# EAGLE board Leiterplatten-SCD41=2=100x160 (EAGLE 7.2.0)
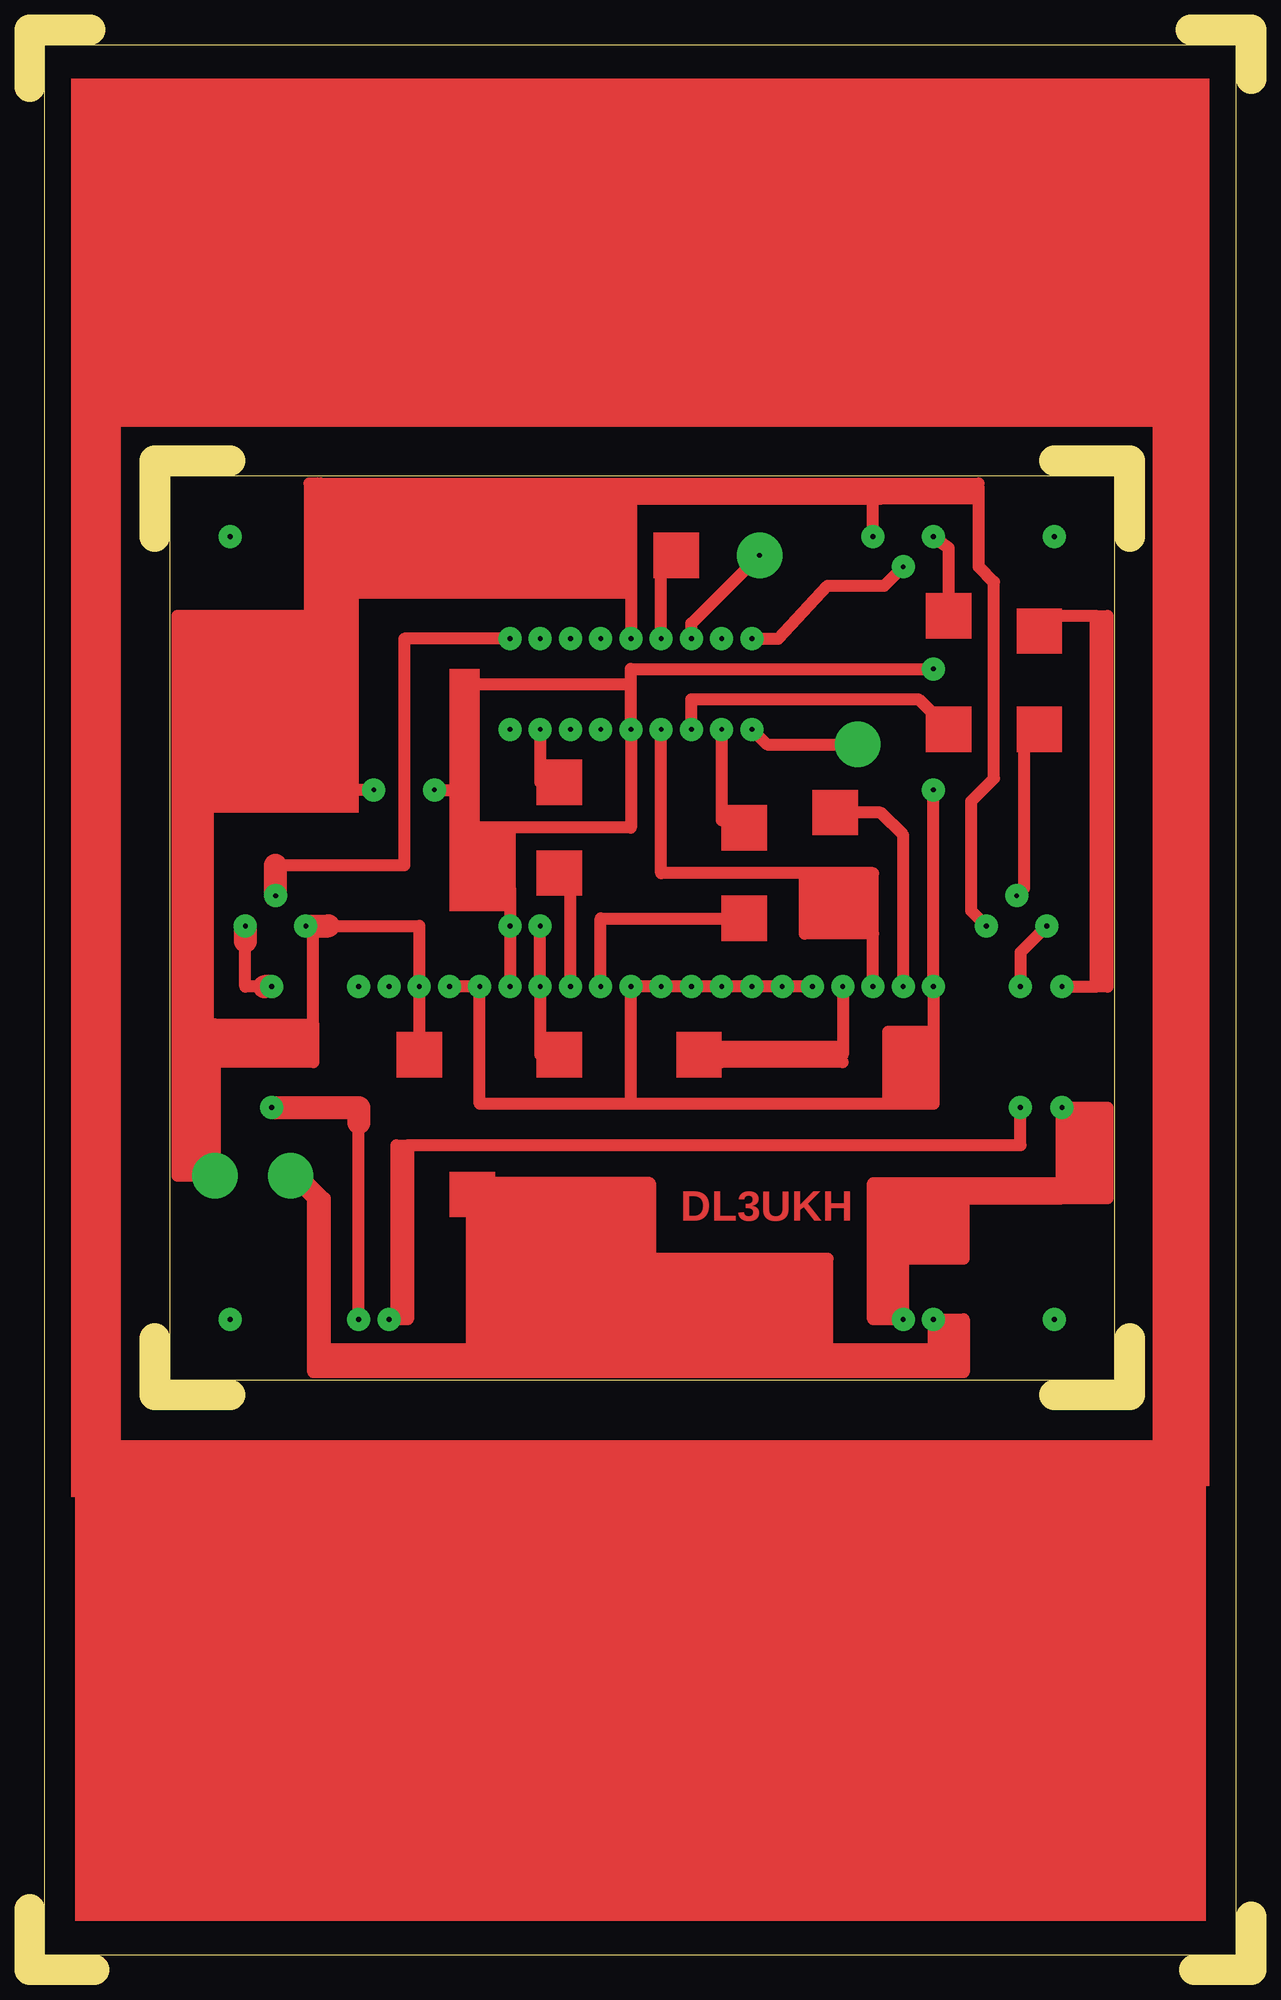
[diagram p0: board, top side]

Size 102.55 x 162.88 mm. Coordinates in mm from the lower left corner, seen from the top.
Outline: 5.4,0 0.32,0
Outline: 0,0 0,5.08
Outline: 97.79,0 102.55,0 102.55,4.45
Outline: 5.08,162.88 0,162.88 0,158.12
Outline: 102.55,158.75 102.55,162.88
Outline: 97.47,162.88 102.23,162.88
Outline: 10.48,120.33 10.48,126.68 16.83,126.68
Outline: 10.48,53.02 10.48,48.26 16.83,48.26
Outline: 86.04,48.26 92.39,48.26 92.39,53.02
Outline: 92.39,120.33 92.39,126.68 86.04,126.68
Outline: 1.27,1.27 101.28,1.27 101.28,161.61 1.27,161.61 1.27,1.27
Outline: 11.75,125.41 11.75,49.53 91.12,49.53 91.12,125.41 11.75,125.41
Copper layers (1*16): Top 0.035mm / dielectric 1.5mm / Bottom 0.035mm
Design rules "default": minimum track width 10mil, minimum drill 24mil, track to track 8mil, track to pad 8mil, pad to pad 8mil, via to via 8mil, smd to smd 8mil, copper to edge 40mil, drill to drill 8mil, minimum pad ring 10mil, minimum via ring 8mil, stop-mask expansion 4mil, vias tented up to drill 0mil, thermal gap 10mil

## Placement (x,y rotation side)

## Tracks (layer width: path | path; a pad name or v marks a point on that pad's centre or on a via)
S$1  (via drill 0.4 pad 1.93)
  Top 1.016: v33.97,99.06 36.51,99.06
S$2  (via drill 0.4 pad 1.93)
  other vias: 60.64,82.55
S$3  (via drill 0.4 pad 1.93)
  Top 1.016: v55.56,104.14 55.56,106.68 74.61,106.68 77.15,104.14
S$4  (via drill 0.4 pad 1.93)
  Top 1.016: v58.1,104.14 58.1,96.52 60.01,96.52
S$5  (via drill 0.4 pad 1.93)
  Top 1.016: v42.86,104.14 42.86,99.69 44.45,99.69
S$6  (via drill 0.4 pad 1.93)
  Top 1.016: v80.33,87.63 79.06,88.9 79.06,98.11 80.96,100.01 80.96,116.52 79.69,117.79 79.69,123.51 | 79.69,123.51 79.69,124.46 70.8,124.46 | 24.13,120.33 24.13,123.51 | 24.13,123.51 24.13,124.46 | 24.13,124.46 24.45,124.46 | 24.45,124.46 50.48,124.46 | 50.48,124.46 50.48,123.51 | 50.48,123.51 50.48,115.57 | 50.48,115.57 v50.48,111.76 | 50.48,124.46 58.42,124.46 | 58.42,124.46 70.8,124.46 | v70.8,120.33 70.8,124.46 | 58.42,124.46 71.44,123.51 | 24.13,124.46 24.13,124.78 | 24.13,124.78 24.45,124.78 | 24.45,124.78 79.69,124.78 | 50.48,123.51 24.13,123.51 | 50.48,123.51 71.44,123.51 | 79.69,123.51 71.44,123.51 | 24.45,124.46 24.45,124.78 | 24.13,124.78 23.5,124.78 23.5,112.39 | 50.48,115.57 23.81,115.57
S$7  (via drill 0.4 pad 1.93)
  other vias: 42.86,111.76
S$8  (via drill 0.4 pad 1.93)
  other vias: 86.04,54.61
S$9  (via drill 0.4 pad 1.93)
  other vias: 86.04,120.33
S$10  (via drill 0.01 pad 3.81, 0.4 pad 1.93)
  Top 1.016: v55.56,111.76 55.56,113.03 v61.28,118.74 | v60.64,104.14 61.91,102.87 v69.53,102.87 | v73.34,82.55 73.34,95.25 71.44,97.16 67.63,97.16
S$11  (via drill 0.4 pad 1.93)
  other vias: 58.1,82.55
S$12  (via drill 0.4 pad 1.93)
  Top 1.016: 31.75,69.21 83.19,69.21 v83.19,72.39 | 31.75,69.21 31.75,54.61 30.8,54.61 | 30.8,54.61 v30.16,54.61 | 30.8,54.61 30.8,69.21 31.75,69.21
S$13  (via drill 0.4 pad 1.93)
  other vias: 75.88,109.22
S$14  (via drill 0.4 pad 1.93)
  Top 1.016: v47.94,82.55 47.94,88.27 60.01,88.27
S$15  (via drill 0.4 pad 1.93)
  Top 1.016: v68.26,82.55 68.26,77.47 | 68.26,77.47 68.26,76.83 57.15,76.83 | 68.26,77.47 57.47,77.47
S$16  (via drill 0.4 pad 1.93)
  Top 1.016: v75.88,120.33 77.15,119.38 77.15,113.66
S$17  (via drill 0.4 pad 1.93)
  Top 1.016: v82.87,90.17 83.5,90.8 83.5,103.5
S$18  (via drill 0.4 pad 1.93)
  Top 1.016: 78.74,64.77 86.68,64.77 | 73.34,66.04 70.8,66.04 70.8,54.61 v73.34,54.61 73.34,59.69 | 73.34,66.04 78.42,66.04 | 78.42,66.04 86.68,66.04 | 86.68,66.04 v86.68,72.39 90.49,72.39 90.49,64.77 86.68,64.77 | 73.34,59.69 73.34,66.04 | 78.42,65.41 78.42,59.69 73.34,59.69 | 78.42,65.41 78.42,66.04 | 86.68,64.77 86.68,65.41 | 86.68,66.04 86.68,65.41 | 86.68,65.41 78.42,65.41
S$19  (via drill 0.4 pad 1.93)
  Top 1.016: v27.62,54.61 27.62,71.12
  Top 1.93: v20.32,72.39 27.62,72.39 27.62,71.12
S$20  (via drill 0.4 pad 1.93)
  Top 1.016: v28.89,99.06 24.77,99.06
S$21  (via drill 0.4 pad 1.93)
  other vias: 58.1,111.76
S$22  (via drill 0.4 pad 1.93)
  other vias: 40.32,104.14
S$23  (via drill 0.4 pad 1.93)
  Top 1.016: v75.88,99.06 v75.88,82.55 75.88,78.74 | 75.88,78.74 75.88,72.71 72.07,72.71 | 72.07,72.71 50.48,72.71 | v65.72,82.55 v63.18,82.55 v55.56,82.55 v50.48,82.55 50.48,72.71 | v35.24,82.55 v37.78,82.55 37.78,72.71 50.48,72.71 | 75.88,78.74 72.07,78.74 72.07,72.71
S$24  (via drill 0.4 pad 1.93)
  Top 1.016: v45.4,82.55 45.4,91.12
S$25  (via drill 0.4 pad 1.93)
  other vias: 30.16,82.55
S$26  (via drill 0.4 pad 1.93)
  other vias: 27.62,82.55
S$27  (via drill 0.4 pad 1.93)
  Top 1.016: v86.68,82.55 89.53,82.55 | 89.53,82.55 89.53,113.66 | 89.53,113.66 83.5,113.66 | 89.53,113.66 90.49,113.66 90.49,82.55 89.53,82.55
S$28  (via drill 0.01 pad 3.81, 0.4 pad 1.93)
  Top 1.016: 37.47,66.04 52.07,66.04 52.07,59.69 | 75.88,52.07 v75.88,54.61 78.42,54.61 78.42,50.8 | 75.88,52.07 75.88,50.8 | 75.88,50.8 37.15,50.8 | 37.15,50.8 37.15,59.69 | 37.15,59.69 37.15,65.09 | 37.15,50.8 23.81,50.8 | 23.81,50.8 23.81,52.07 | 23.81,52.07 23.81,64.77 | 23.81,64.77 v21.91,66.67 | 78.42,50.8 75.88,50.8 | 75.88,52.07 23.81,52.07 | 78.42,50.8 78.42,50.17 23.81,50.17 23.81,50.8 | 66.99,51.44 66.99,59.69 52.07,59.69 | 52.07,59.69 37.15,59.69 | 23.81,64.77 24.77,64.77 | 24.77,64.77 24.77,51.44 | 24.77,64.77 22.22,67.31
S$29  (via drill 0.4 pad 1.93)
  other vias: 16.83,54.61
S$30  (via drill 0.4 pad 1.93)
  Top 1.016: v40.32,111.76 31.43,111.76 31.43,92.71 20.64,92.71
  Top 1.93: v20.64,90.17 20.64,92.71
S$31  (via drill 0.4 pad 1.93)
  Top 1.016: v60.64,111.76 62.87,111.76 66.99,116.2 71.75,116.2 v73.34,117.79
S$32  (via drill 0.01 pad 3.81, 0.4 pad 1.93)
  Top 1.016: 24.13,113.66 24.13,110.49 14.92,110.49 | 24.13,113.66 14.92,113.66 | 14.92,113.66 12.38,113.66 12.38,79.38 | 14.92,113.66 14.92,110.49 | 12.38,79.38 12.38,66.67 v15.56,66.67 15.56,79.38 | 14.92,110.49 14.92,79.38 | 14.92,79.38 12.38,79.38 | 15.24,76.2 23.81,76.2 23.81,79.38 | 14.92,79.38 15.56,79.38 | 15.56,79.38 23.81,79.38 | 23.81,79.38 23.81,86.99 v23.18,87.63 | 25.08,87.63 32.7,87.63 v32.7,82.55 32.7,77.15 | 24.13,113.66 24.13,115.89
  Top 1.93: v23.18,87.63 25.08,87.63
S$33  (via drill 0.4 pad 1.93)
  Top 1.016: 19.68,82.55 18.1,82.55 18.1,86.36
  Top 1.93: v18.1,87.63 18.1,86.36 | v20.32,82.55 19.68,82.55
S$34  (via drill 0.4 pad 1.93)
  other vias: 16.83,120.33
S$35  (via drill 0.4 pad 1.93)
  Top 1.016: v42.86,87.63 v42.86,82.55 42.86,76.83
S$36
  Top 1.016: 68.26,76.2 58.1,76.2
S$37  (via drill 0.4 pad 1.93)
  other vias: 47.94,104.14
S$38  (via drill 0.4 pad 1.93)
  other vias: 45.4,111.76
S$39  (via drill 0.4 pad 1.93)
  Top 1.016: v53.02,111.76 53.02,117.47 54.61,117.47 54.61,119.06
S$40  (via drill 0.01 pad 3.81)
  other vias: 61.28,118.74 69.53,102.87 21.91,66.67 15.56,66.67
S$41  (via drill 0.4 pad 1.93)
  other vias: 47.94,111.76
S$42  (via drill 0.4 pad 1.93)
  Top 1.016: v85.41,87.63 83.19,85.41 v83.19,82.55
S$43
  Top 1.016: 24.77,120.33 24.77,123.83
S$44  (via drill 0.4 pad 1.93)
  Top 1.016: v70.8,82.55 70.8,86.99 | 70.8,86.99 70.8,92.08 65.09,92.08 | 65.09,92.08 53.02,92.08 v53.02,104.14 | 70.8,86.99 65.09,86.99 65.09,92.08
S$45  (via drill 0.4 pad 1.93)
  other vias: 45.4,104.14
S$46  (via drill 0.4 pad 1.93)
  Top 1.016: 40.32,95.88 50.48,95.88 v50.48,104.14 50.48,107.95 | 40.32,95.88 37.15,95.88 40.32,90.8 | v40.32,82.55 v40.32,87.63 40.32,90.8 | 50.48,107.95 50.48,109.22 75.88,109.22 | 40.32,90.8 37.15,90.8 | 35.88,107.95 50.48,107.95 | 40.32,90.8 40.32,95.88
S$48  (via drill 0.4 pad 1.93)
  other vias: 53.02,82.55
(copper drawn outside any net)
  shapes: Top area x39

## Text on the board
Top: DL3UKH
